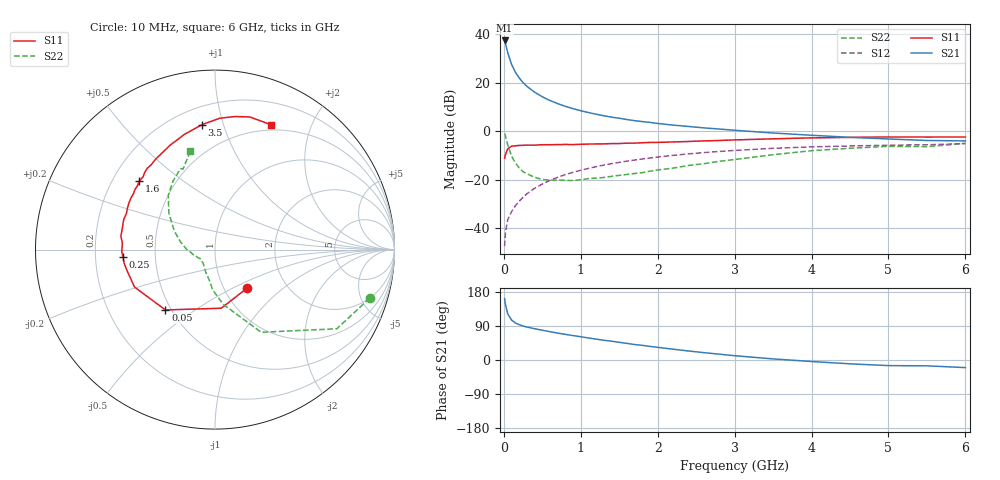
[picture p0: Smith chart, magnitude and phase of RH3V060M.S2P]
! SIEMENS Small Signal Semiconductors
! BFR106
! Si NPN RF Bipolar Junction Transistor in SOT23
! VCE = 3 V  IC = 60 mA
! Common Emitter S-Parameters:  August  1996
# GHz  S  MA  R  50
!  f  S11  S21  S12  S22
! GHz  MAG  ANG  MAG  ANG  MAG  ANG  MAG  ANG
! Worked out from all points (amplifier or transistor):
!   36 points, 10 MHz to 6 GHz, reference 50 ohm
!   highest |S21| = 37.4 dB at 10 MHz (marker M1)
!   |S21| within 3 dB of that: start of sweep to 34.85 MHz
!   unconditionally stable (mu >= 1): 218.3 MHz to 2.463 GHz; 5.46 GHz to 5.83 GHz
!   at 250 MHz: K = 1.03, MAG = 22.6 dB, |S12| = -27.2 dB
!   at 1.4 GHz: K = 1.06, MAG = 8.1 dB, |S12| = -13.3 dB
!   at 6 GHz: K = 1.00, MSG = 0.5 dB, |S12| = -5.1 dB
!   S11 on the Smith chart (normalised r, x): 10 MHz: 1.29, -0.59; 50 MHz: 0.47, -0.39; 250 MHz: 0.32, -0.04; 1.6 GHz: 0.31, +0.35; 3.5 GHz: 0.31, +0.85; 6 GHz: 0.44, +1.45
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0.01  0.2794 -49.7  74.39 161.8  0.0043 80.4  0.9026 -17.5
0.02  0.3285 -83.9  65.83 147.4  0.0081 71.8  0.8096 -33.0
0.05  0.4351 -129.4  41.94 121.9  0.0149 61.6  0.5277 -60.8
0.1  0.4945 -155.0  24.07 105.5  0.0221 62.0  0.3089 -81.4
0.15  0.5027 -165.7  16.49 97.7  0.0293 65.4  0.2239 -93.4
0.2  0.5116 -171.2  12.57 93.1  0.0364 68.7  0.176 -100.1
0.25  0.5142 -175.5  10.08 89.6  0.0439 70.3  0.1471 -107.9
0.3  0.5195 -178.7  8.44 87.0  0.0516 71.8  0.1334 -113.3
0.4  0.5173 175.9  6.393 82.6  0.0668 72.6  0.1127 -122.8
0.5  0.5298 171.9  5.136 78.5  0.0819 72.3  0.1017 -130.0
0.6  0.5293 167.9  4.301 74.7  0.0977 71.4  0.0986 -135.0
0.7  0.5325 164.3  3.717 71.0  0.1129 70.5  0.0986 -140.1
0.9  0.5329 157.9  2.923 64.4  0.143 67.8  0.0964 -149.1
1.1  0.5455 151.5  2.432 58.1  0.1722 65.1  0.1058 -155.0
1.3  0.5508 145.7  2.092 52.1  0.2016 62.0  0.1119 -161.5
1.6  0.569 137.9  1.746 43.8  0.243 57.3  0.1294 -169.9
2.2  0.604 122.8  1.341 28.5  0.3195 47.7  0.1745 173.3
2.8  0.6467 108.9  1.113 15.4  0.3842 38.0  0.2413 156.9
3.5  0.7001 95.9  0.922 2.9  0.4463 27.3  0.3296 141.3
4.5  0.7497 81.5  0.751 -10.1  0.4981 12.8  0.4475 121.5
5.5  0.7608 69.6  0.647 -15.4  0.5279 3.7  0.4831 111.6
6  0.762 65.8  0.634 -20.1  0.5586 -3.2  0.5648 104.1
